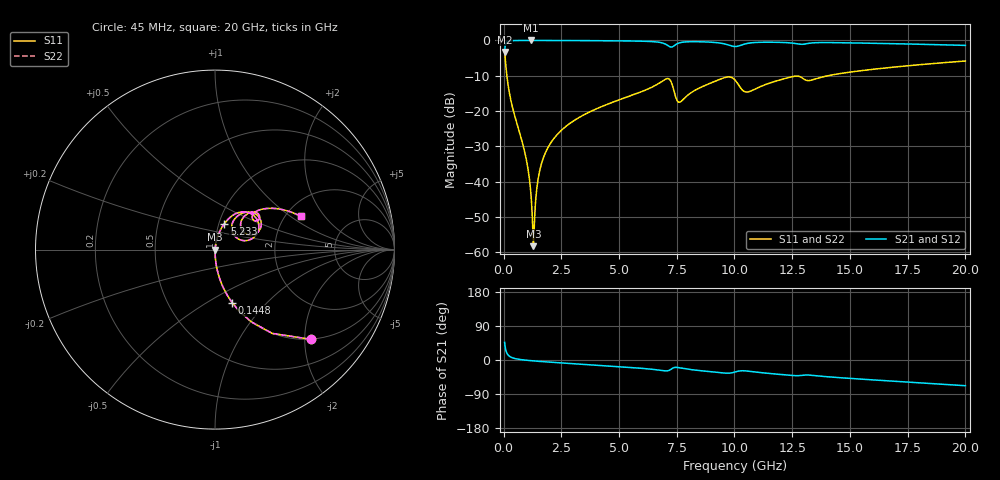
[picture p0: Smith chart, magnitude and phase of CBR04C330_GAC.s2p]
! S-parameter model data by Modelithics Inc.  support@modelithics.com 813-866-6335  Tampa FL USA
! S-Parameter data specifications:
! Substrate: 20-mil Rogers 4350B, substrate thickness, H=0.508mm, Dielectric constant, Er=3.75
! PCB Mounting Pad Footprint: Pad width, PadW=0.52mm , Pad length, PadL=0.52mm , Pad gap, PadG (edge-to-edge)=0.28mm , Reference planes=1.32mm apart
#  GHz  S  MA  R 50
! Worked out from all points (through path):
!   801 points, 45 MHz to 20 GHz, reference 50 ohm
!   highest |S21| = -0.01 dB at 1.167 GHz (marker M1); lowest = -3.3 dB at 45 MHz (marker M2)
!   group delay of S21, straight-line fit = 9.51 ps
!   lowest |S11| = -58.3 dB at 1.292 GHz (marker M3), VSWR 1.00, Z = 50.1 - j0.0196 ohm
!   |S11| at or under -10 dB: 142.7 MHz to 14.05 GHz (13.9 GHz wide, 196 % of centre)
!   |S22| runs from -58.3 to -2.7 dB; largest |S21 - S12| = 0
!   S11 on the Smith chart (normalised r, x): 45 MHz: 1.00, -2.13; 144.8 MHz: 1.00, -0.66; 5.233 GHz: 1.06, +0.31; 20 GHz: 2.39, +1.20
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0.045  0.7299 -43.2  0.6833 46.8  0.6833 46.8  0.7299 -43.2
0.144775  0.3117 -72.0  0.9497 17.9  0.9497 17.9  0.3117 -72.0
0.344325  0.1287 -83.0  0.991 6.8  0.991 6.8  0.1287 -83.0
0.967919  0.02198 -87.8  0.9987 -0.5  0.9987 -0.5  0.02198 -87.8
1.167469  0.007806 -83.2  0.9988 -1.7  0.9988 -1.7  0.007806 -83.2
1.217356  0.004742 -77.6  0.9988 -2.0  0.9988 -2.0  0.004742 -77.6
1.292188  0.001223 -9.2  0.9987 -2.4  0.9987 -2.4  0.001223 -9.2
1.367019  0.004244 70.1  0.9987 -2.8  0.9987 -2.8  0.004244 70.1
1.541625  0.01317 80.6  0.9985 -3.6  0.9985 -3.6  0.01317 80.6
1.865894  0.028 81.9  0.9981 -5.1  0.9981 -5.1  0.028 81.9
3.387462  0.08522 77.5  0.9942 -11.2  0.9942 -11.2  0.08522 77.5
5.2333  0.1534 70.1  0.9843 -18.5  0.9843 -18.5  0.1534 70.1
6.704981  0.2442 57.6  0.9447 -26.4  0.9447 -26.4  0.2442 57.6
7.178913  0.2827 30.9  0.8208 -27.1  0.8208 -27.1  0.2827 30.9
7.6279  0.1336 39.2  0.926 -20.7  0.926 -20.7  0.1336 39.2
9.249244  0.2717 50.1  0.9287 -32.7  0.9287 -32.7  0.2717 50.1
10.0225  0.2754 24.3  0.8195 -31.7  0.8195 -31.7  0.2754 24.3
10.54632  0.1857 35.5  0.9058 -29.1  0.9058 -29.1  0.1857 35.5
12.54182  0.3088 42.0  0.9135 -41.0  0.9135 -41.0  0.3088 42.0
13.36496  0.276 41.3  0.9223 -40.5  0.9223 -40.5  0.276 41.3
16.68248  0.4121 33.6  0.9019 -55.2  0.9019 -55.2  0.4121 33.6
20  0.5114 21.3  0.8506 -67.8  0.8506 -67.8  0.5114 21.3
